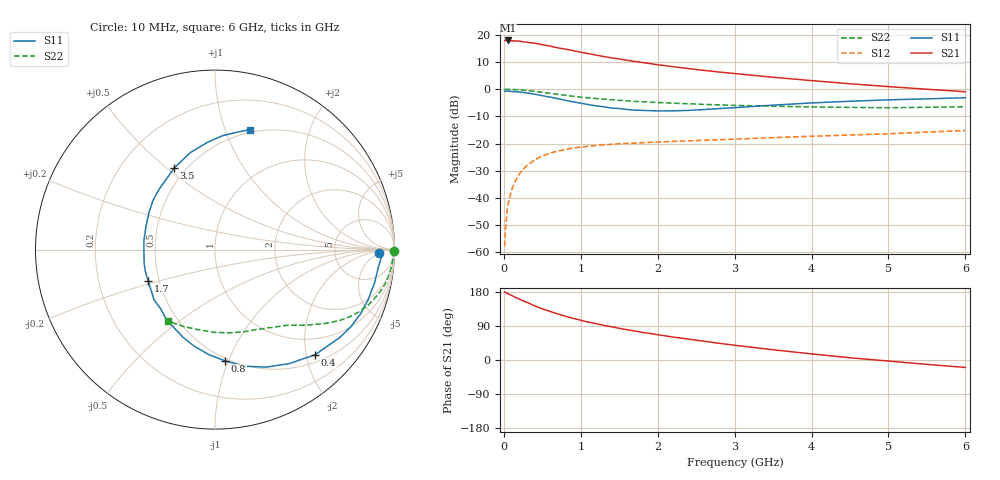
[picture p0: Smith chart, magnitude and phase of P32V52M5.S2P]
! SIEMENS Small Signal Semiconductors
! BFP181
! Si NPN RF Bipolar Junction Transistor in SOT143
! VCE = 2.5 V  IC = 2.5 mA
! Common Emitter S-Parameters:  March  1996
# GHz  S  MA  R  50
!  f  S11  S21  S12  S22
! GHz  MAG  ANG  MAG  ANG  MAG  ANG  MAG  ANG
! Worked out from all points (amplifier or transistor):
!   36 points, 10 MHz to 6 GHz, reference 50 ohm
!   highest |S21| = 17.9 dB at 50 MHz (marker M1)
!   |S21| within 3 dB of that: start of sweep to 760.9 MHz
!   unconditionally stable (mu >= 1): 2.226 GHz to end of sweep
!   at 250 MHz: K = 0.14, MSG = 23.4 dB, |S12| = -29.5 dB
!   at 1.4 GHz: K = 0.72, MSG = 15.9 dB, |S12| = -20.3 dB
!   at 6 GHz: K = 1.12, MAG = 5.1 dB, |S12| = -15.2 dB
!   S11 on the Smith chart (normalised r, x): 10 MHz: 21, -6; 400 MHz: 0.64, -2.17; 800 MHz: 0.48, -0.97; 1.7 GHz: 0.43, -0.18; 3.5 GHz: 0.43, +0.53; 6 GHz: 0.47, +1.22
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0.01  0.9161 -1.3  7.813 179.1  0.0013 85.9  0.9954 -0.5
0.02  0.9285 -2.5  7.84 178.5  0.0026 85.7  0.9883 -1.0
0.05  0.916 -5.9  7.844 175.1  0.0072 88.7  0.992 -2.7
0.1  0.9078 -12.0  7.722 170.4  0.0139 81.9  0.9882 -5.4
0.2  0.8861 -23.9  7.636 160.7  0.0273 75.9  0.9712 -10.6
0.25  0.8704 -29.6  7.401 156.2  0.0336 72.9  0.9571 -13.2
0.3  0.8503 -35.1  7.293 152.3  0.0395 69.5  0.943 -15.3
0.4  0.8089 -46.4  6.986 143.0  0.05 63.6  0.9101 -19.7
0.5  0.7576 -57.0  6.56 135.0  0.0592 57.9  0.8726 -23.5
0.6  0.7137 -66.6  6.174 128.2  0.0667 53.5  0.837 -26.6
0.7  0.6699 -75.8  5.739 121.6  0.0727 49.4  0.8019 -29.4
0.8  0.6221 -84.9  5.437 115.5  0.0778 46.0  0.7698 -31.6
1  0.5512 -102.0  4.754 104.8  0.0859 40.4  0.7142 -35.5
1.1  0.5199 -110.1  4.497 100.0  0.0893 38.0  0.6909 -37.1
1.4  0.4476 -132.4  3.758 87.6  0.0969 32.7  0.6381 -41.4
1.7  0.411 -155.2  3.232 76.5  0.1018 29.6  0.5966 -45.0
2.2  0.3997 172.3  2.582 60.5  0.1094 25.9  0.5526 -51.0
2.8  0.4397 142.1  2.061 44.0  0.1177 23.1  0.5145 -59.2
3.5  0.5077 116.7  1.651 27.0  0.1284 20.5  0.4857 -70.4
4.5  0.5987 94.1  1.254 5.9  0.1435 16.7  0.4613 -90.3
5.5  0.6631 79.9  0.996 -11.6  0.1624 13.9  0.4628 -112.0
6  0.6953 73.9  0.895 -19.6  0.1735 11.3  0.4751 -123.1
